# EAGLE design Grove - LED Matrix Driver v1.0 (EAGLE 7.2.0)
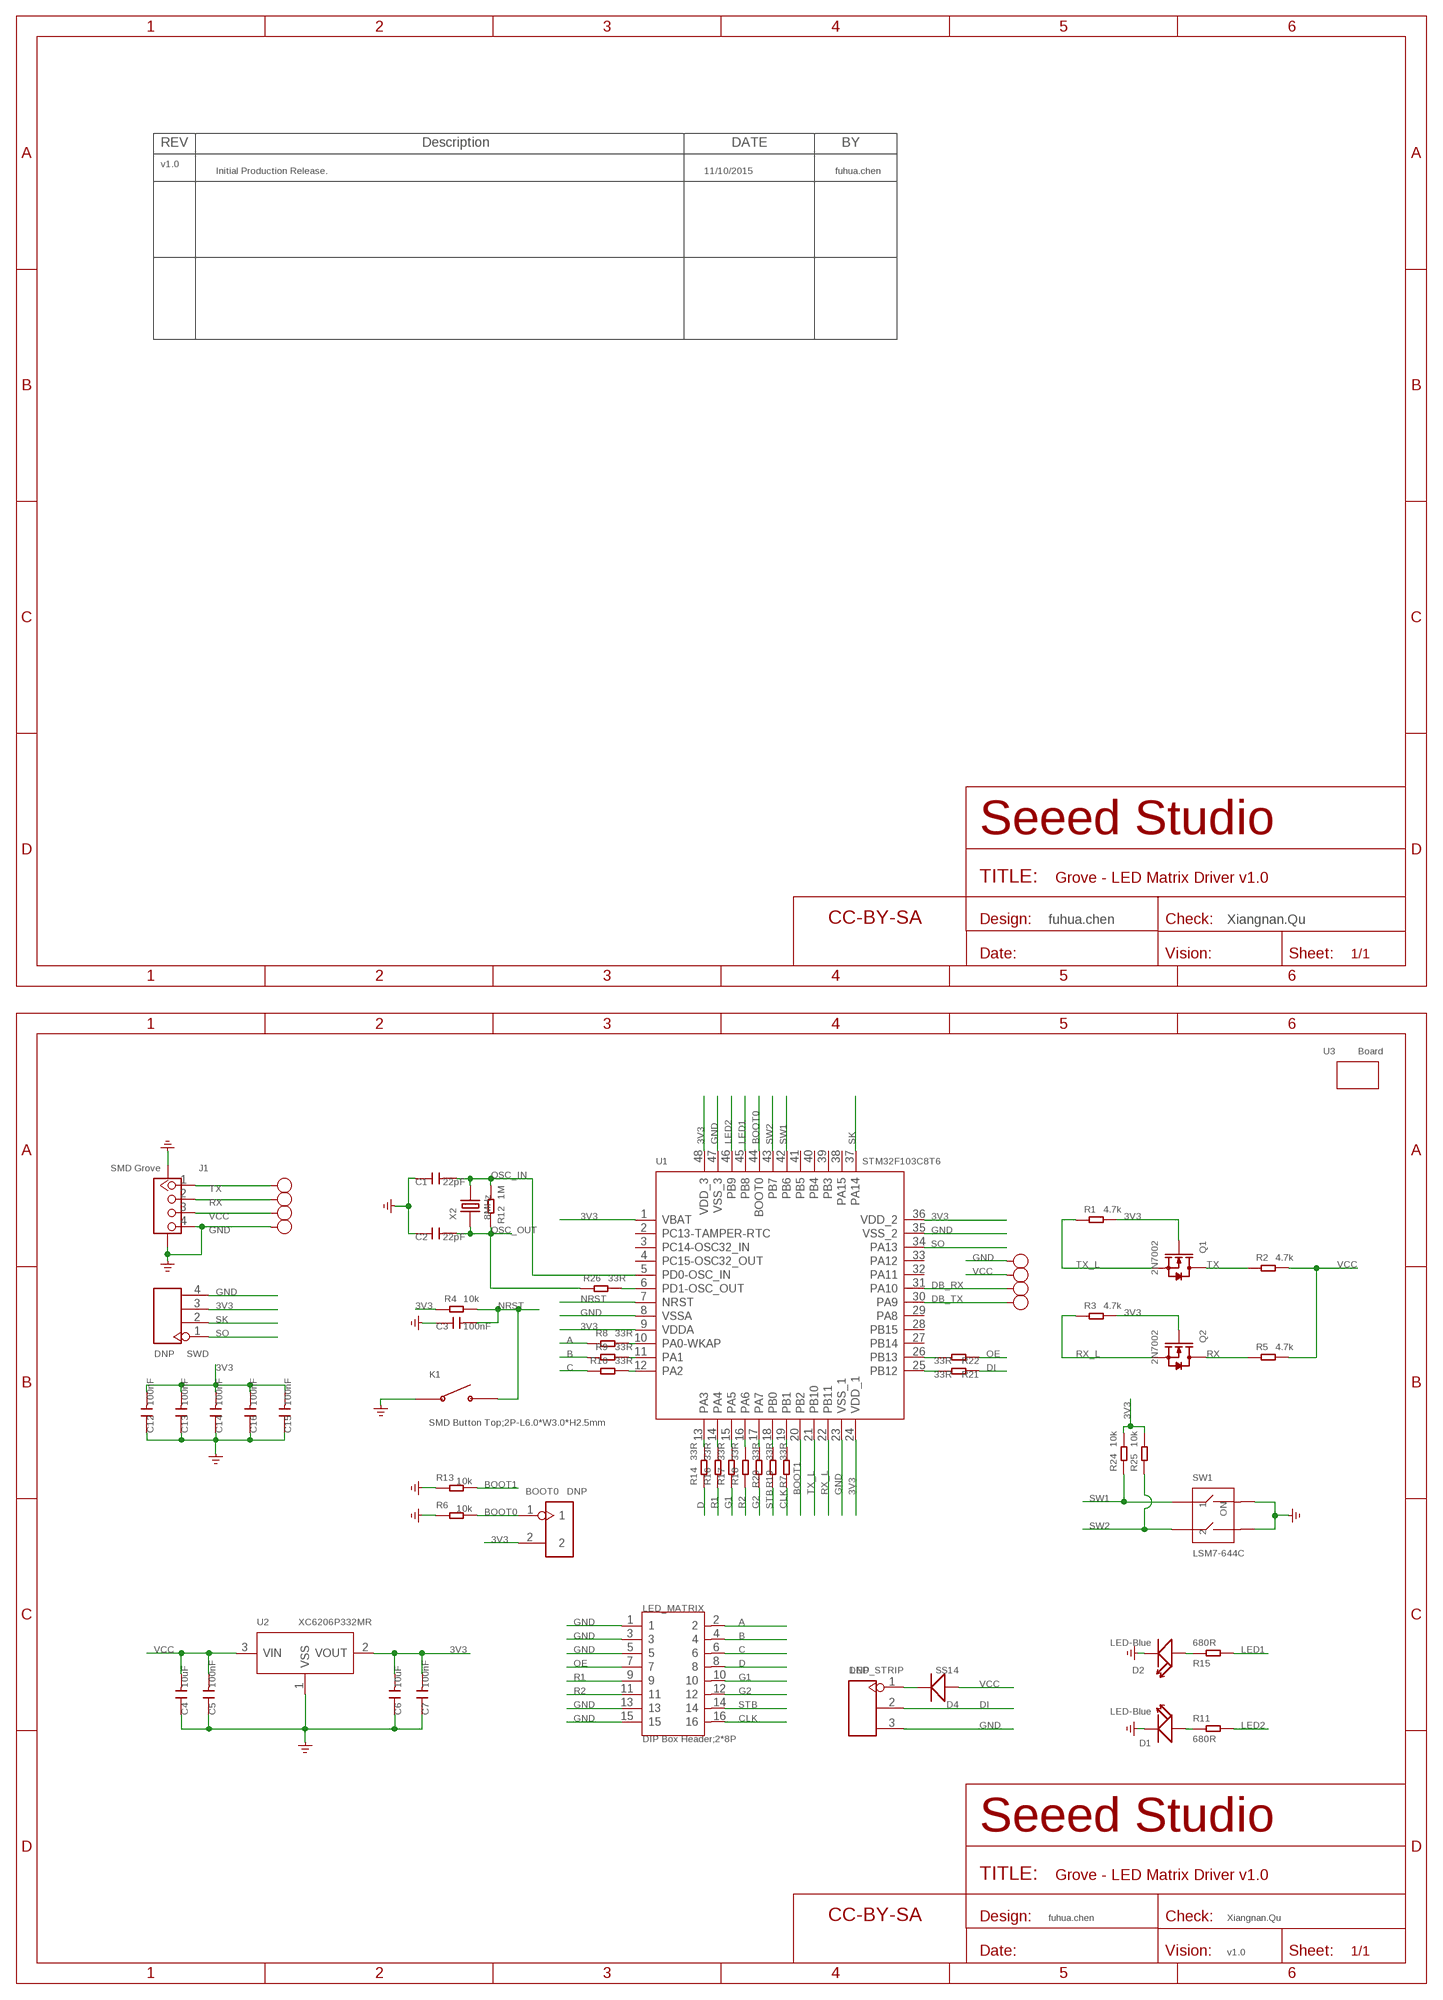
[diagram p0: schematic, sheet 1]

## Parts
BOOT0  DNP  HEADER-2P-1.5  [H2-1.5]
C1  22pF  CAP-0402  [C0402]
C2  22pF  CAP-0402  [C0402]
C3  100nF  CAP-0402  [C0402]
C4  10uF  CAP-0402  [C0402]
C5  100nF  CAP-0402  [C0402]
C6  10uF  CAP-0402  [C0402]
C7  100nF  CAP-0402  [C0402]
C12  100nF  CAP-0402  [C0402]
C13  100nF  CAP-0402  [C0402]
C14  100nF  CAP-0402  [C0402]
C15  100nF  CAP-0402  [C0402]
C16  100nF  CAP-0402  [C0402]
D1  LED-Blue  LED-0402  [LED-0402]
D2  LED-Blue  LED-0402  [LED-0402]
D4  SS14  DIODE'SMA'  [DO-214AC]
DB_RX  RX  TEST-POINT'4545'  [TP-D45MIL]
DB_TX  TX  TEST-POINT'4545'  [TP-D45MIL]
FR  FR2  SEEEDSTUDIO-OPEN-SCH-FRAME  [SEEEDSTUDIO-PCB-FRAME]
FR1  FR1  SEEEDSTUDIO-OPEN-SCH-FRAME  [SEEEDSTUDIO-PCB-FRAME]
GND  GND  TEST-POINT'4545'  [TP-D45MIL]
GND13  GND  TEST-POINT'4545'  [TP-D45MIL]
J1  SMD Grove  GROVE-CONNECTOR-SMD'90D'  [HW4-SMD-2.0-90D]
K1  SMD Button Top;2P-L6.0*W3.0*H2.5mm  BUTTON-2P-SMD  [SW2-SMD-6.0X3.0X2.5MM]
LED_MATRIX  DIP Box Header;2*8P  HEADER-2X8P  [H2X8_2.54]
LED_STRIP  DNP  HEADER-3P-2.54  [H3-2.54]
Q1  2N7002  MOSFET-N'SOT23'  [SOT-23]
Q2  2N7002  MOSFET-N'SOT23'  [SOT-23]
R1  4.7k  RES-0402  [R0402]
R2  4.7k  RES-0402  [R0402]
R3  4.7k  RES-0402  [R0402]
R4  10k  RES-0402  [R0402]
R5  4.7k  RES-0402  [R0402]
R6  10k  RES-0402  [R0402]
R7  33R  RES-0402  [R0402]
R8  33R  RES-0402  [R0402]
R9  33R  RES-0402  [R0402]
R10  33R  RES-0402  [R0402]
R11  680R  RES-0402  [R0402]
R12  1M  RES-0402  [R0402]
R13  10k  RES-0402  [R0402]
R14  33R  RES-0402  [R0402]
R15  680R  RES-0402  [R0402]
R16  33R  RES-0402  [R0402]
R17  33R  RES-0402  [R0402]
R18  33R  RES-0402  [R0402]
R19  33R  RES-0402  [R0402]
R20  33R  RES-0402  [R0402]
R21  33R  RES-0402  [R0402]
R22  33R  RES-0402  [R0402]
R24  10k  RES-0402  [R0402]
R25  10k  RES-0402  [R0402]
R26  33R  RES-0402  [R0402]
RX  RX  TEST-POINT'4545'  [TP-D45MIL]
SW1  LSM7-644C  SWITCHES-2X2P'KM-02'  [SW4-SMD-2.54-5.08X6.8X3.3MM]
SWD  DNP  HEADER-4P-65/35MIL  [H4-2.54]
TX  TX  TEST-POINT'4545'  [TP-D45MIL]
U1  STM32F103C8T6  MCU-STM32F103CBT6  [LQFP48]
U2  XC6206P332MR  PMIC-XC6206PMR  [SOT-23]
U3  Board  GROVE'2X2U'  [GROVE-2*2-DRILL-DIM]
VCC  VCC  TEST-POINT'4545'  [TP-D45MIL]
VCC1  VCC  TEST-POINT'4545'  [TP-D45MIL]
X2  8MHz  CRYSTAL-2P'5032'  [X2-SMD-5.0X3.2X1.3MM]

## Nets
3V3: BOOT0.2 C6.2 C7.2 C12.2 C13.2 C14.2 C15.2 C16.2 Q1.1(G) Q2.1(G) R1.2 R3.2 R4.1 R24.2 R25.2 SWD.3 U1.1(VBAT) U1.9(VDDA) U1.24(VDD_1) U1.36(VDD_2) U1.48(VDD_3) U2.2(VOUT)
A: LED_MATRIX.2 R8.1
B: LED_MATRIX.4 R9.1
BOOT0: BOOT0.1 R6.2 U1.44(BOOT0)
BOOT1: R13.2 U1.20(PB2)
C: LED_MATRIX.6 R10.1
CLK: LED_MATRIX.16 R7.2
D: LED_MATRIX.8 R14.1
DB_RX: DB_RX.T U1.31(PA10)
DB_TX: DB_TX.T U1.30(PA9)
DI: LED_STRIP.2 R21.2
G1: LED_MATRIX.10 R17.1
G2: LED_MATRIX.12 R20.2
GND: C1.1 C2.1 C3.1 C4.1 C5.1 C6.1 C7.1 C12.1 C13.1 C14.1 C15.1 C16.1 D1.- D2.- GND13.T GND.T J1.4 J1.SS1 J1.SS2 K1.1 LED_MATRIX.1 LED_MATRIX.3 LED_MATRIX.5 LED_MATRIX.13 LED_MATRIX.15 LED_STRIP.3 R6.1 R13.1 SW1.3 SW1.4 SWD.4 U1.8(VSSA) U1.23(VSS_1) U1.35(VSS_2) U1.47(VSS_3) U2.1(VSS) ; supply symbol labelled GND_POWER
LED1: R15.2 U1.45(PB8)
LED2: R11.2 U1.46(PB9)
N$1: D1.+ R11.1
N$2: R19.1 U1.18(PB0)
N$3: R9.2 U1.11(PA1)
N$4: D2.+ R15.1
N$5: R14.2 U1.13(PA3)
N$6: R16.2 U1.14(PA4)
N$7: R17.2 U1.15(PA5)
N$8: R18.2 U1.16(PA6)
N$9: R10.2 U1.12(PA2)
N$10: R8.2 U1.10(PA0-WKAP)
N$11: R7.1 U1.19(PB1)
N$12: R20.1 U1.17(PA7)
N$14: R22.1 U1.26(PB13)
N$15: R21.1 U1.25(PB12)
N$16: R26.2 U1.6(PD1-OSC_OUT)
N$17: D4.2(-) LED_STRIP.1
NRST: C3.2 K1.P$2 R4.2 U1.7(NRST)
OE: LED_MATRIX.7 R22.2
OSC_IN: C1.2 R12.2 U1.5(PD0-OSC_IN) X2.2
OSC_OUT: C2.2 R12.1 R26.1 X2.1
R1: LED_MATRIX.9 R16.1
R2: LED_MATRIX.11 R18.1
RX: J1.2 Q2.3(D) R5.1 RX.T
RX_L: Q2.2(S) R3.1 U1.22(PB11)
SK: SWD.2 U1.37(PA14)
SO: SWD.1 U1.34(PA13)
STB: LED_MATRIX.14 R19.2
SW1: R24.1 SW1.1 U1.42(PB6)
SW2: R25.1 SW1.2 U1.43(PB7)
TX: J1.1 Q1.3(D) R2.1 TX.T
TX_L: Q1.2(S) R1.1 U1.21(PB10)
VCC: C4.2 C5.2 D4.1(+) J1.3 R2.2 R5.2 U2.3(VIN) VCC1.T VCC.T
Unconnected: U1.2(PC13-TAMPER-RTC) U1.3(PC14-OSC32_IN) U1.4(PC15-OSC32_OUT) U1.27(PB14) U1.28(PB15) U1.29(PA8) U1.32(PA11) U1.33(PA12) U1.38(PA15) U1.39(PB3) U1.40(PB4) U1.41(PB5)

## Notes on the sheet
- REV | Description | DATE | BY
- v1.0
- Initial Production Release. | 11/10/2015 | fuhua.chen
- fuhua.chen | Xiangnan.Qu
- D1
- fuhua.chen | Xiangnan.Qu
- v1.0

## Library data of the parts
BOOT0 = Connector-new:HEADER-2P
C1-C7 C12-C16 = Discrete-new:CAP: Ceramic Capacitors
D1 D2 = Discrete-new:LED
D4 = Discrete-new:DIODE*
DB_RX DB_TX GND GND13 RX TX VCC VCC1 = Discrete-new:TEST-POINT; PARTNO: DNP
FR FR1 = moudle-new:SEEEDSTUDIO-OPEN-SCH-FRAME
J1 = Connector-new:GROVE-CONNECTOR-SMD: 4P-SMD-2.0:320110030;4P-SMD-2.0-90D:320110032
K1 = Discrete-new:BUTTON-2P: SW2-3.4X6.0X3.55MM-90D:311020025;SW2-SMD-6.0X3.0X2.5MM:311020029
LED_MATRIX = Connector-new:HEADER-2X8P
LED_STRIP = Connector-new:HEADER-3P
Q1 Q2 = Discrete-new:MOSFET-N
R1-R22 R24-R26 = Discrete-new:RES
SW1 = Discrete-new:SWITCHES-2X2P
SWD = Connector-new:HEADER-4P
U1 = IC-new:MCU-STM32F103CBT6: 310010004
U2 = IC-new:PMIC-XC6206P: LOW ESR Cap.Compatible Positive Voltage Regulators
U3 = moudle-new:GROVE
X2 = Discrete-new:CRYSTAL-2P

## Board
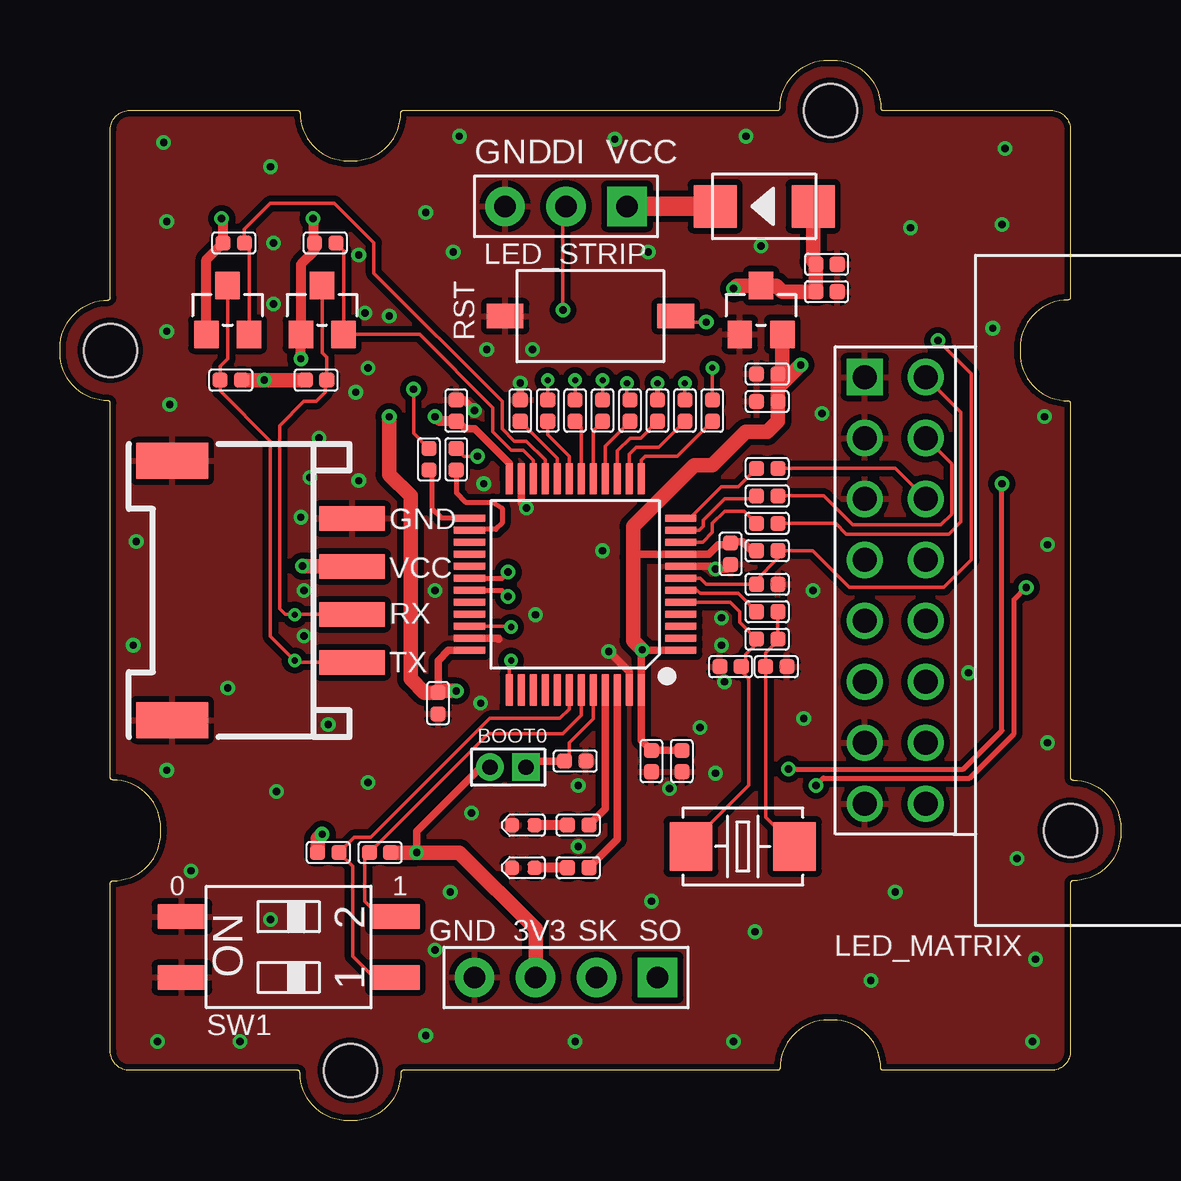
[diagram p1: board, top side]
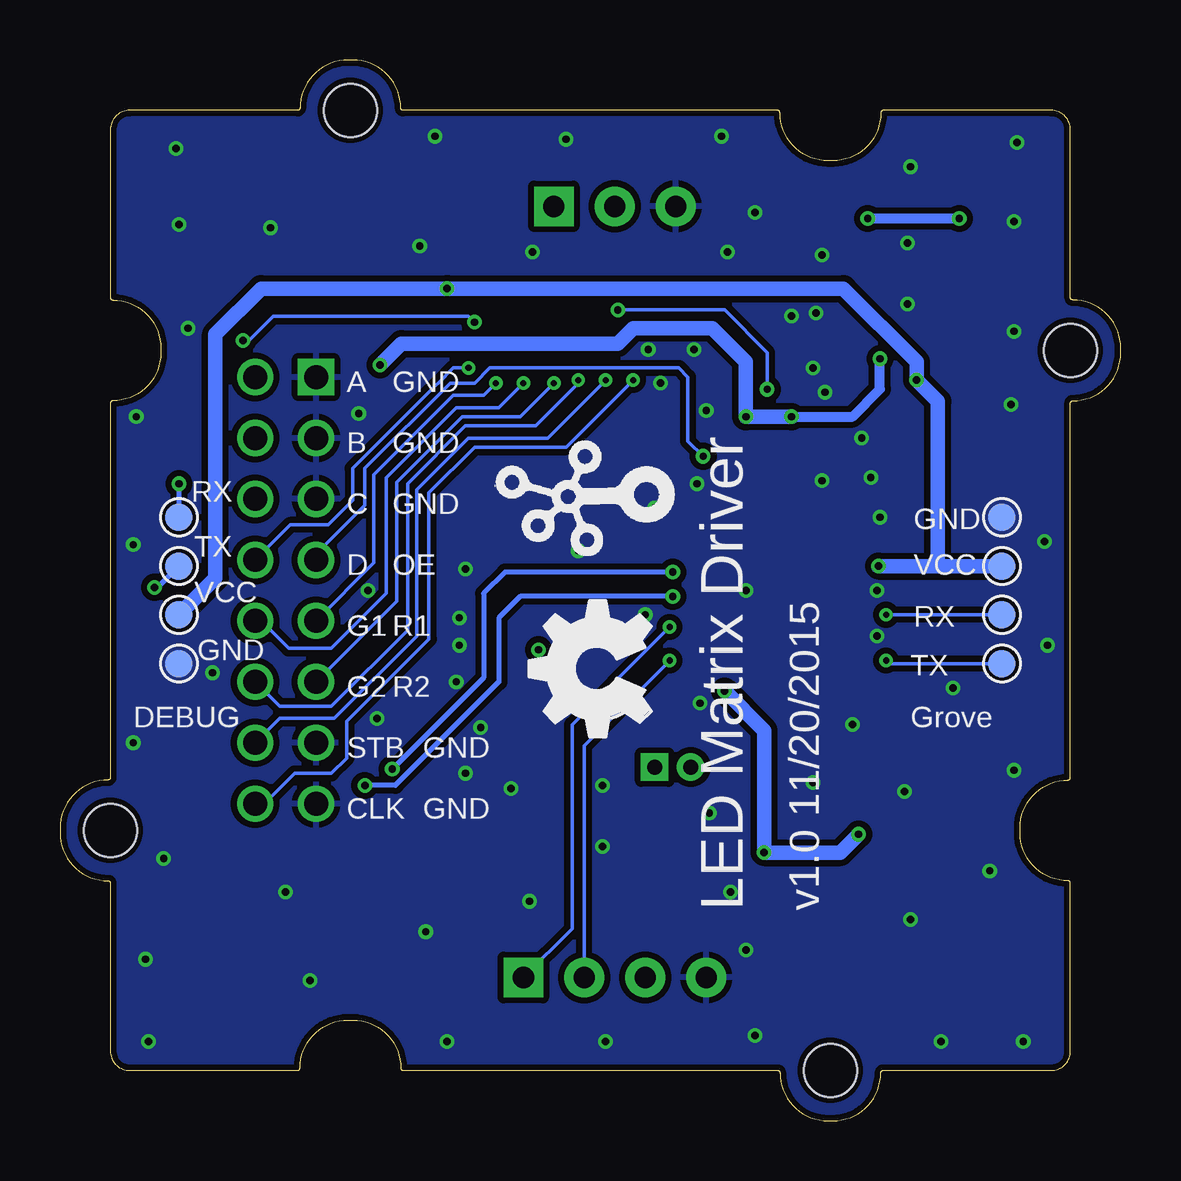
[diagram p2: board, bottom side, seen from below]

Size 44.2 x 44.2 mm. Coordinates in mm from the lower left corner, seen from the top.
Copper layers (1*16): Top 0.035mm / dielectric 1.5mm / Bottom 0.035mm
Design rules "SeeedStudio_2layer_DRU_no_angle_20140221 *": minimum track width 6mil, minimum drill 10mil, track to track 6mil, track to pad 6mil, pad to pad 6mil, via to via 6mil, smd to smd 0mil, copper to edge 10mil, drill to drill 10mil, minimum pad ring 10mil, minimum via ring 6mil, stop-mask expansion 2mil, vias tented up to drill 25mil, thermal gap 10mil

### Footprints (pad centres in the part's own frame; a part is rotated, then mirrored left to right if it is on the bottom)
H2-1.5 = drill 0.635 pad 1.016 square: 1 0,0.75 | drill 0.635 pad 1.016: 2 0,-0.75
C0402 = smd 0.635 x 0.635: 1 0,0.445; 2 0,-0.445
LED-0402 = smd 0.58 x 0.58: + -0.468,0; - 0.468,0
DO-214AC = smd 1.8 x 1.77: 1 -2.042,0; 2 2.042,0
TP-D45MIL = smd 1.143 x 1.143: T 0,0
HW4-SMD-2.0-90D = smd 1.01 x 2.74: 1 -3,-0.1; 2 -1,-0.1; 3 1,-0.1; 4 3,-0.1 | smd 1.5 x 3: SS1 -5.4,7.4; SS2 5.4,7.4
SW2-SMD-6.0X3.0X2.5MM = smd 1.524 x 1.016: 1 -3.556,0; P$2 3.556,0
H2X8_2.54 = drill 1 square: 1 -1.27,8.89 | drill 1: 2 1.27,8.89; 3 -1.27,6.35; 4 1.27,6.35; 5 -1.27,3.81; 6 1.27,3.81; 7 -1.27,1.27; 8 1.27,1.27; 9 -1.27,-1.27; 10 1.27,-1.27; 11 -1.27,-3.81; 12 1.27,-3.81; 13 -1.27,-6.35; 14 1.27,-6.35; 15 -1.27,-8.89; 16 1.27,-8.89
H3-2.54 = drill 0.889 pad 1.651 square: 1 0,2.54 | drill 0.889 pad 1.651: 2 0,0; 3 0,-2.54
SOT-23 = smd 1.016 x 1.143: 1 -0.889,-1.016; 2 0.889,-1.016; 3 0,1.016
R0402 = smd 0.635 x 0.635: 1 0,0.445; 2 0,-0.445
SW4-SMD-2.54-5.08X6.8X3.3MM = smd 1.016 x 2.032: 1 -1.27,-4.445; 2 1.27,-4.445; 3 1.27,4.445; 4 -1.27,4.445
H4-2.54 = drill 0.889 pad 1.651 square: 1 0,3.81 | drill 0.889 pad 1.651: 2 0,1.27; 3 0,-1.27; 4 0,-3.81
LQFP48 = smd 1.3 x 0.3: 1 -4.4,2.75; 2 -4.4,2.25; 3 -4.4,1.75; 4 -4.4,1.25; 5 -4.4,0.75; 6 -4.4,0.25; 7 -4.4,-0.25; 8 -4.4,-0.75; 9 -4.4,-1.25; 10 -4.4,-1.75; 11 -4.4,-2.25; 12 -4.4,-2.75; 25 4.4,-2.75; 26 4.4,-2.25; 27 4.4,-1.75; 28 4.4,-1.25; 29 4.4,-0.75; 30 4.4,-0.25; 31 4.4,0.25; 32 4.4,0.75; 33 4.4,1.25; 34 4.4,1.75; 35 4.4,2.25; 36 4.4,2.75 | smd 0.3 x 1.3: 13 -2.75,-4.4; 14 -2.25,-4.4; 15 -1.75,-4.4; 16 -1.25,-4.4; 17 -0.75,-4.4; 18 -0.25,-4.4; 19 0.25,-4.4; 20 0.75,-4.4; 21 1.25,-4.4; 22 1.75,-4.4; 23 2.25,-4.4; 24 2.75,-4.4; 37 2.75,4.4; 38 2.25,4.4; 39 1.75,4.4; 40 1.25,4.4; 41 0.75,4.4; 42 0.25,4.4; 43 -0.25,4.4; 44 -0.75,4.4; 45 -1.25,4.4; 46 -1.75,4.4; 47 -2.25,4.4; 48 -2.75,4.4
GROVE-2*2-DRILL-DIM = hole 2.2: 10,20; -20,10; -10,-20; 20,-10
X2-SMD-5.0X3.2X1.3MM = smd 1.778 x 2.032: 1 -2.159,0; 2 2.159,0

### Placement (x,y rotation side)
BOOT0  18.67,14.73 270 top
C1  27.94,18.93 90 top
C2  29.85,18.93 270 top
C3  29.47,22.35 270 top
C4  31.94,34.55 270 top
C5  31.94,35.69 270 top
C6  29.47,29.97 90 top
C7  29.47,31.12 90 top
C12  27.94,23.62 180 top
C13  16.51,29.59 0 top
C14  25.91,14.99 180 top
C15  24.64,14.99 180 top
C16  15.75,17.4 180 top
D1  19.31,10.54 180 top
D2  19.31,12.32 180 top
D4  29.34,38.1 180 top
DB_RX  39.25,23.12 0 bottom
DB_TX  39.25,25.15 0 bottom
FR  not placed on the board
FR1  not placed on the board
GND  4.96,25.15 90 bottom
GND13  39.25,19.05 0 bottom
J1  12.07,22.1 90 top
K1  22.1,33.53 0 top
LED_MATRIX  34.8,22.1 0 top
LED_STRIP  21.08,38.1 270 top
Q1  6.99,33.78 0 top
Q2  10.92,33.78 0 top
R1  7.24,36.58 270 top
R2  7.11,30.86 90 top
R3  11.05,36.58 270 top
R4  29.47,23.75 90 top
R5  10.67,30.86 270 top
R6  21.46,14.99 270 top
R7  20.32,29.59 180 top
R8  29.47,24.89 270 top
R9  29.47,26.04 270 top
R10  29.47,27.18 270 top
R11  21.59,10.54 90 top
R12  29.47,20.07 270 top
R13  19.18,29.59 0 top
R14  27.18,29.59 0 top
R15  21.59,12.32 90 top
R16  26.04,29.59 0 top
R17  24.89,29.59 0 top
R18  23.75,29.59 0 top
R19  21.46,29.59 180 top
R20  22.61,29.59 180 top
R21  15.37,27.56 180 top
R22  16.51,27.56 180 top
R24  11.18,11.18 270 top
R25  13.34,11.18 90 top
R26  29.47,21.21 270 top
RX  4.96,21.08 90 bottom
SW1  9.53,7.24 90 top
SWD  21.08,5.97 270 top
TX  4.96,19.05 90 bottom
U1  21.46,22.35 180 top
U2  29.21,33.78 0 top
U3  22.1,22.1 0 top
U$3  [OSHW_FILLX200_NOTEXT]  19.56,16 90 bottom
U$8  [GROVE-SILK-BIG]  19.56,26.04 90 bottom
VCC  4.96,23.12 90 bottom
VCC1  39.25,21.08 0 bottom
X2  28.45,11.43 180 top

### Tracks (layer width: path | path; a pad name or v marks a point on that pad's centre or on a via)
3V3  (via drill 0.3, 0.3 pad 0.46)
  Top 0.305: U1.24 18.72,27.39 17.27,28.83 16.89,28.83 16.58,29.15 C13.2 | 26.04,15.56 C14.2 C15.2 24.22,15.86 U1.48 24.22,19.54 24.28,19.6 | U1.36 16.18,19.6 15.75,19.18 C16.2 | R4.1 28.83,23.75 28.45,24.13 28.01,24.13 C12.2 27.88,24.01 27.43,24.01 27.03,23.6 U1.9 23.99,23.6 23.88,23.5 | U1.1 24.28,19.6 | 24.28,19.6 v24.26,19.62 | BOOT0.2 17.53,14.73 14.86,12.07 v14.86,11.18
  Top 0.406: Q1.1 6.1,35.88 R1.2 6.8,37.53 v6.73,37.59 | v10.54,37.59 10.54,36.64 R3.2 10.61,36.26 10.04,35.69 Q2.1 v10.04,31.75 | C13.2 15.81,29.15 v15.62,29.34
  Top 0.61: v16.51,17.91 15.81,17.91 C16.2 15.18,17.85 14.61,18.42 14.61,26.04 13.72,26.93 v13.72,29.34 | R25.2 v14.86,11.18 16.64,11.18 19.81,8 SWD.3 | R24.2 10.73,11.75 v10.92,11.94 | C6.2 C7.2 30.1,31.31 U2.2 | C6.2 29.91,30.55 v30.86,31.5 | C6.2 29.91,29.15 29.47,28.7 28.58,28.7 27.18,27.31 26.42,27.31 23.88,24.77 23.88,23.5 23.88,20.01 v24.26,19.62
  Bottom 0.406: v6.73,37.59 v10.54,37.59 | v13.72,29.34 11.18,29.34 10.04,30.48 v10.04,31.75
  Bottom 0.61: v10.92,11.94 11.69,11.18 v14.86,11.18 14.86,16.26 v16.51,17.91 | v30.86,31.5 29.97,32.39 20.96,32.39 20.32,33.02 17.02,33.02 15.62,31.62 v15.62,29.34 v13.72,29.34
A
  Top 0.152: R8.1 32.32,24.89 32.77,24.45 37.02,24.45 37.53,24.96 37.53,29.53 LED_MATRIX.2
B
  Top 0.152: R9.1 31.82,26.04 33.02,24.83 36.7,24.83 37.15,25.28 37.15,27.37 LED_MATRIX.4
BOOT0
  Top 0.152: U1.44 22.21,16.75 21.21,15.75 21.21,15.18 R6.2
  Top 0.305: R6.2 19.68,14.99 BOOT0.1
BOOT1
  Top 0.152: U1.20 20.71,27.61 R13.2
C
  Top 0.152: R10.1 34.8,27.18 LED_MATRIX.6
CLK  (via drill 0.25)
  Top 0.152: v20.32,30.86 R7.2
  Bottom 0.152: LED_MATRIX.16 35.69,13.21 34.42,14.48 32.9,14.48 32.26,15.12 32.26,16.64 28.83,20.07 28.83,26.16 26.93,28.07 23.12,28.07 v20.32,30.86
D  (via drill 0.25)
  Top 0.152: R14.1 v27.18,31.37
  Bottom 0.152: LED_MATRIX.8 34.61,24.83 33.02,24.83 32.01,25.85 32.01,27.18 28.51,30.67 28.45,30.74 27.82,31.37 v27.18,31.37
DB_RX  (via drill 0.3 pad 0.46)
  Top 0.203: U1.31 18.41,22.1 v18.67,21.85 | v40.26,22.23 39.75,21.72 39.75,16.13 37.9,14.28 31.8,14.28 v31.5,13.97
  Bottom 0.203: v18.67,21.85 25.02,21.85 25.91,20.96 25.91,18.29 30.23,13.97 v31.5,13.97 | v40.26,22.23 40.13,22.23 DB_RX.T
DB_TX  (via drill 0.3 pad 0.46)
  Top 0.203: U1.30 18.41,22.6 v18.67,22.86 | v30.36,14.66 37.65,14.66 39.25,16.26 v39.25,26.55
  Bottom 0.203: v18.67,22.86 25.66,22.86 26.55,21.97 26.55,18.47 v30.36,14.66 | v39.25,26.55 DB_TX.T
DI  (via drill 0.3)
  Top 0.152: v14.73,30.48 14.73,28.64 R21.2 | v20.96,33.78 20.96,37.98 LED_STRIP.2
  Bottom 0.152: v20.96,33.78 16.51,33.78 14.73,32.01 v14.73,30.48
G1  (via drill 0.25)
  Top 0.203: v24.89,30.74 R17.1
  Bottom 0.152: LED_MATRIX.10 35.82,20.83 34.67,19.69 32.9,19.69 30.61,21.97 30.61,26.8 27.69,29.72 25.91,29.72 v24.89,30.74
G2  (via drill 0.25 pad 0.3)
  Top 0.152: R20.2 v22.61,30.86
  Bottom 0.152: 22.61,30.74 24.39,28.96 27.31,28.96 29.72,26.55 29.72,20.45 32.9,17.27 35.05,17.27 LED_MATRIX.12
  Bottom 0.203: v22.61,30.86 22.61,30.74
GND  (via drill 0.3, 0.3 pad 0.46)
  Top 0.305: U1.23 19.22,25.75 v19.43,25.53 | R13.1 v19.18,30.74 | 16.51,30.1 C13.1 16.83,30.04 v17.27,29.59 | U1.35 18.25,20.1 18.29,20.07 | C12.1 27.75,22.99 v27.31,22.99 27.19,23.1 U1.8 | U1.47 23.71,18.71 v22.86,19.56
  other vias: 27.56,19.81 27.56,20.96 31.37,22.1 30.99,16.77 27.31,14.48 26.67,16.39 27.69,18.29 25.4,13.85 34.8,9.53 28.96,7.88 21.59,13.97 10.04,25.15 10.42,26.8 12.45,26.67 17.66,26.55 19.81,21.08 24.64,9.15 17.15,12.83 40.52,3.3 28.07,3.3 41.15,24.01 15.62,7.11 16.26,9.53 8.77,8.38 5.46,10.42 4.07,3.3 7.5,3.3 15.24,3.56 21.46,3.3 12.83,14.1 11.18,16.51 17.53,17.4 9.02,13.72 6.99,18.04 4.57,29.85 4.45,32.9 12.83,31.37 12.32,30.36 10.8,28.45 8.89,36.58 8.89,34.04 15.24,37.85 4.32,40.77 4.45,37.47 8.77,39.75 16.64,41.02 23.12,40.9 28.58,41.02 29.21,36.45 24.51,36.2 16.39,36.2 17.78,32.13 19.69,32.13 12.7,33.66 13.72,33.53 12.45,36.07 22.61,23.75 31.75,29.47 41.02,29.34 41.15,15.75 39.37,40.52 35.44,37.21 39.25,37.34 21.59,11.43 33.78,5.84 40.64,6.73 39.88,10.92 3.18,24.13 3.05,19.81 38.86,33.02 15.62,22.1 37.85,18.67 10.16,22.1 10.16,20.2 4.45,14.61
  pour Bottom (isolate 0.254): 2.8,44.71 40.64,44.71 44.07,41.28 44.07,14.86 44.83,14.1 44.83,2.16 41.53,-1.14 0.26,-1.14 -5.97,5.08 -5.97,35.94
  pour Top (isolate 0.254): 3.69,45.34 41.53,45.34 44.96,41.91 44.96,15.5 45.72,14.73 45.72,2.8 42.42,-0.51 1.15,-0.51 -5.08,5.72 -5.08,36.58
  pour Bottom (isolate 0.254): 2.8,44.71 40.64,44.71 44.07,41.28 44.07,14.86 44.83,14.1 44.83,2.16 41.53,-1.14 0.26,-1.14 -5.97,5.08 -5.97,35.94
LED1
  Top 0.305: U1.45 22.71,13 R15.2
LED2
  Top 0.305: U1.46 23.21,11.72 R11.2
N$1
  Top 0.406: R11.1 D1.+
N$2
  Top 0.152: U1.18 21.71,28.9 R19.1
N$3
  Top 0.152: U1.11 26.64,24.6 26.8,24.77 26.8,25.02 27.69,25.91 28.9,25.91 R9.2
N$4
  Top 0.406: R15.1 D2.+
N$5
  Top 0.152: U1.13 24.22,27.52 24.39,27.69 25.72,27.69 R14.2
N$6
  Top 0.152: U1.14 23.71,27.78 24.01,28.07 24.96,28.07 R16.2
N$7
  Top 0.152: U1.15 23.21,27.91 23.75,28.45 24.2,28.45 R17.2
N$8
  Top 0.152: U1.16 22.71,28.11 R18.2
N$9
  Top 0.152: U1.12 26.25,25.1 27.56,26.42 28.26,26.42 R10.2
N$10
  Top 0.152: U1.10 26.77,24.1 27.18,24.51 27.18,24.89 27.69,25.4 28.51,25.4 R8.2
N$11
  Top 0.152: U1.19 21.21,27.68 20.32,28.58 R7.1
N$12
  Top 0.152: U1.17 22.21,28.76 R20.1
N$14
  Top 0.203: R22.1 16.51,26.16 16.89,25.78 18.04,25.78 18.42,25.53 18.42,24.89 18.16,24.64 17.1,24.64 U1.26
N$15
  Top 0.203: R21.1 15.5,27.12 15.5,25.53 15.9,25.12 17.05,25.12 U1.25
N$16
  Top 0.152: 28.77,21.46 R26.2 28.26,21.97 26.67,21.97 26.54,22.1 U1.6
N$17
  Top 0.813: D4.2 LED_STRIP.1
NRST  (via drill 0.3)
  Top 0.152: v36.58,32.51 37.98,31.12 37.98,23.37 36.83,22.23 32.9,22.23 31.37,23.75 R4.2 29.91,23.43 29.02,22.55 C3.2 26.93,22.35 26.68,22.6 U1.7 | v26.93,33.28 25.91,33.28 K1.P$2
  Bottom 0.152: v36.58,32.51 36.32,32.51 35.31,33.53 27.18,33.53 v26.93,33.28
OE  (via drill 0.3 pad 0.3)
  Top 0.152: v17.4,27.69 16.83,27.69 R22.2
  Bottom 0.152: LED_MATRIX.7 33.53,23.62 31.5,25.66 31.5,27.18 27.94,30.74 26.93,30.74 26.29,31.37 18.42,31.37 18.04,30.99 18.04,28.32 v17.4,27.69
OSC_IN
  Top 0.152: U1.5 27.93,21.6 28.32,21.21 28.32,20.77 R12.2 29.02,19.88 28.58,19.43 28.58,19.12 C1.2 28.39,18.73 28.7,18.42 28.7,13.97 26.29,11.56 X2.2
OSC_OUT
  Top 0.152: R26.1 R12.1 29.91,20.01 29.4,19.5 C2.2 29.4,12.64 X2.1
R1  (via drill 0.25)
  Top 0.152: v26.04,30.74 R16.1
  Bottom 0.152: v26.04,30.74 26.55,30.23 27.82,30.23 31.12,26.93 31.12,23.24 LED_MATRIX.9
R2  (via drill 0.25)
  Top 0.152: v23.62,30.74 23.62,30.16
  Top 0.203: 23.62,30.16 23.75,30.16 R18.1
  Bottom 0.152: v23.62,30.74 25.02,29.34 27.43,29.34 30.16,26.61 30.16,21.66 LED_MATRIX.11
RX  (via drill 0.25)
  Top 0.152: J1.2 9.8,21.1 | 9.8,21.1 v9.78,21.08 | 9.8,21.1 9.38,21.1 9.15,21.34 9.15,28.96 10.16,29.97 10.67,29.97 11.05,30.36 11.05,30.8 R5.1 11.11,31.82 10.92,32.01 Q2.3
  Bottom 0.152: RX.T v9.78,21.08
RX_L
  Top 0.152: R3.1 11.81,36.26 Q2.2 14.99,32.77 18.04,29.72 18.04,28.7 18.8,27.94 19.31,27.94 19.72,27.53 U1.22
SK  (via drill 0.25)
  Top 0.152: U1.37 18.72,19.1 v18.8,19.18
  Bottom 0.152: 18.67,19.05 v18.8,19.18 22.35,15.62 SWD.2
SO  (via drill 0.25)
  Top 0.152: U1.34 18.77,20.6 v18.8,20.58
  Bottom 0.152: v18.8,20.58 19.31,20.07 19.43,19.94 22.86,16.51 22.86,8 SWD.1
STB  (via drill 0.25)
  Top 0.152: v21.46,30.86 R19.2
  Bottom 0.152: LED_MATRIX.14 35.05,16.77 32.77,16.77 29.34,20.2 29.34,26.29 27.18,28.45 23.88,28.45 v21.46,30.86
SW1
  Top 0.152: U1.42 21.21,17.15 20.83,16.77 17.91,16.77 12.96,11.81 12.26,11.81 R24.1 12.19,10.61 12.19,6.86 13.08,5.97 SW1.1
SW2
  Top 0.152: U1.43 21.71,16.89 20.96,16.13 17.85,16.13 R25.1 12.7,10.99 12.7,9.15 13.34,8.51 SW1.2
TX  (via drill 0.25)
  Top 0.152: Q1.3 6.99,31.75 6.67,31.44 R2.1 6.67,30.42 8.77,28.32 8.77,20.2 v9.78,19.18 9.86,19.1 J1.1
  Bottom 0.152: TX.T 9.65,19.05 v9.78,19.18
TX_L
  Top 0.152: Q1.2 7.88,36.39 R1.1 7.69,37.15 8.77,38.23 11.43,38.23 13.08,36.58 13.08,35.31 18.42,29.97 18.42,28.83 18.93,28.32 19.43,28.32 20.21,27.54 U1.21
VCC  (via drill 0.3)
  Top 0.61: R2.2 v8.51,30.86 R5.2 | D4.1 31.38,35.81 C5.2 C4.2 30.1,34.55 29.85,34.8 U2.3 28.2,34.8 v28.07,34.67 | J1.3 10.11,23.1 v10.1,23.12
  Bottom 0.61: v10.1,23.12 7.88,23.12 | 7.88,23.12 VCC.T | 7.88,23.12 7.62,23.37 7.62,29.97 v8.51,30.86 8.51,31.62 11.56,34.67 v28.07,34.67 35.82,34.67 37.72,32.77 37.72,22.61 VCC1.T

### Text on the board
tPlace: GND | DI | VCC | RST | GND | VCC | RX | TX | 0 | 1 | GND | 3V3 | SK | SO
bPlace: GND | A | GND | B | RX | GND | C | OE | D | TX | VCC | R1 | G1 | GND | R2 | G2 | Grove | DEBUG | GND | STB | GND | CLK | v1.0 11/20/2015 | LED Matrix Driver

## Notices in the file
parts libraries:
moudle-new: This work is licensed under the Creative Commons Attribution 4.0 International License.
To view a copy of this license,visit:
http://creativecommons.org/licenses/by-sa/4.0
moudle-new: CC-BY-SA
